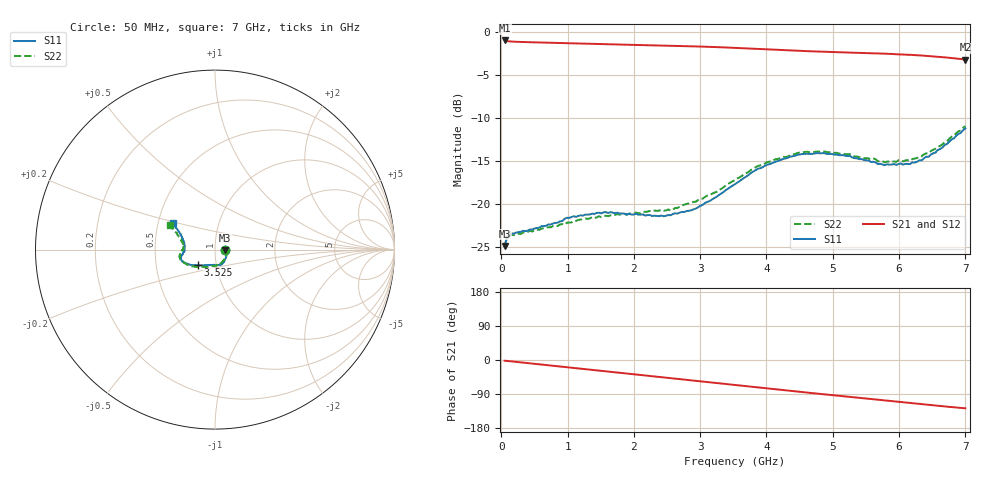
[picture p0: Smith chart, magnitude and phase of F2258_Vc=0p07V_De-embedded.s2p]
! Integrated Device Technology
! Corporate Headquarters
! 6024 Silver Creek Valley Road
! San Jose, CA 95138  USA
! Phone:  1-408-284-8200
! Toll Free:  1-800-223-1366
! Webpage:  http://www.idt.com/
! Timing and RF Division
! 515 Groton Road, Suite 102
! Westford, MA 01886-6024
! Device:  F2258
! Description: Voltage Variable RF Attenuator
! Frequency:  50.0 -  6000.00 MHz
! Package:  3x3 mm Thin QFN Plastic Package: 16 pin
! Ports:  2 RF, 2 DC
!  Pin  1  = NC
!  Pin  2  = NC
!  Pin  3  = RF2  = Port 2
!  Pin  4  = GND
!  Pin  5  = Vdd
!  Pin  6  = NC
!  Pin  7  = VCTRL
!  Pin  8  = NC
!  Pin  9  = GND
!  Pin 10  = RF1  = Port 1
!  Pin 11  = NC
!  Pin 12  = NC
!  Pin 13  = NC
!  Pin 14  = NC
!  Pin 15  = NC
!  Pin 16  = NC
! Vcntrl:  0.070 Volts
! Vdd:  +3.300 Volts
! Current:  1.074 mA
! Data:  The device was measured on a the F2258 evaluation board which has
!  individual transmission lines to the RF pins.  Data was collected
!  using a calibrated network analyzer.  The evaluation board was
!  de-embedded using a TRL calibration technique.
!  The reference plane is the edge of the package pin.
! Misc:  SN 10
!  Action Tracker AT0285
! Date Measured:  2014-12-10
! Date:  2016-01-13  MJV
! Note:
!  Integrated Device Technology supplies this data as a sample of measured
!  data at the package pin for this product.  Your particular data for this
!  product may vary.
!  Data was taken at 25 degrees C.
!  Integrated Device Technology reserves the right to change this data at anytime.
!Freq_(GHz)  S11M_(dB)  S11P_(deg)  S21M_(dB)  S21P_(deg)  S12M_(dB)  S12P_(deg)  S22M_(dB)  S22P_(deg)
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# GHz S dB R 50
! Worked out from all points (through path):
!   201 points, 50 MHz to 7 GHz, reference 50 ohm
!   highest |S21| = -0.96 dB at 50 MHz (marker M1); lowest = -3.2 dB at 7 GHz (marker M2)
!   group delay of S21, straight-line fit = 50.5 ps
!   lowest |S11| = -24.9 dB at 50 MHz (marker M3), VSWR 1.12, Z = 56 - j0.389 ohm
!   |S11| at or under -10 dB: start of sweep to end of sweep
!   |S22| runs from -24.9 to -10.9 dB; largest |S21 - S12| = 0.00041
!   S11 on the Smith chart (normalised r, x): 50 MHz: 1.12, -0.01; 3.525 GHz: 0.81, -0.14; 7 GHz: 0.60, +0.19
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0.05  -24.87 -3.5  -0.96 -1.9  -0.96 -1.9  -24.91 -3.0
0.08475  -23.90 -6.0  -1.03 -2.4  -1.03 -2.5  -23.98 -5.4
0.15425  -23.42 -9.3  -1.08 -3.6  -1.08 -3.6  -23.59 -9.4
0.71025  -22.38 -37.2  -1.22 -14.1  -1.22 -14.1  -22.69 -38.6
0.98825  -21.60 -51.0  -1.27 -19.3  -1.27 -19.3  -22.18 -54.7
1.2315  -21.35 -59.3  -1.32 -23.8  -1.32 -23.8  -21.80 -63.7
1.6485  -20.94 -71.0  -1.41 -31.4  -1.41 -31.4  -21.32 -76.8
2.37825  -21.42 -92.5  -1.54 -44.8  -1.54 -44.7  -20.78 -94.3
2.552  -21.31 -98.4  -1.57 -48.0  -1.57 -48.0  -20.74 -99.6
2.93425  -20.53 -115.1  -1.65 -55.1  -1.65 -55.1  -19.73 -113.0
3.525  -17.69 -137.8  -1.82 -66.2  -1.82 -66.2  -17.21 -135.6
4.0115  -15.43 -151.4  -2.00 -75.2  -2.00 -75.2  -15.12 -151.0
4.46325  -14.28 -159.8  -2.16 -83.4  -2.16 -83.4  -14.07 -162.1
4.7065  -14.15 -163.1  -2.23 -87.7  -2.23 -87.6  -13.96 -166.3
5.15825  -14.31 -168.5  -2.35 -95.6  -2.35 -95.6  -14.14 -173.1
5.61  -15.08 -175.3  -2.45 -103.5  -2.46 -103.5  -14.71 -179.2
5.6795  -15.35 -176.8  -2.46 -104.6  -2.47 -104.6  -15.03 -179.7
5.85325  -15.41 179.0  -2.52 -107.8  -2.52 -107.8  -15.06 175.7
6.166  -15.35 171.2  -2.63 -113.4  -2.63 -113.3  -14.97 169.8
6.33975  -14.93 164.9  -2.71 -116.5  -2.71 -116.5  -14.43 165.5
6.722  -13.01 153.3  -2.94 -123.1  -2.95 -123.1  -12.71 156.4
7  -11.20 147.9  -3.19 -127.4  -3.19 -127.4  -10.92 151.5
